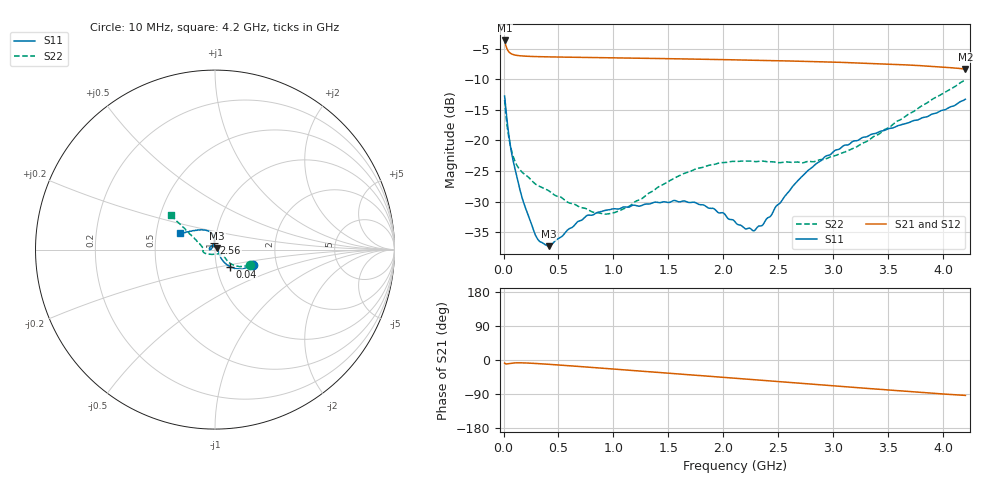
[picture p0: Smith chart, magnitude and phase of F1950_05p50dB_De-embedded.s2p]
! Integrated Device Technology
! Corporate Headquarters
! 6024 Silver Creek Valley Road
! San Jose, CA 95138  USA
! Phone:  1-408-284-8200
! Toll Free:  1-800-223-1366
! Webpage:  http://www.idt.com/
! Timing and RF Division
! 515 Groton Road, Suite 102
! Westford, MA 01886-6024
! Device:  F1950
! Description: 7-bit 0.25 dB Digital Step Attenuator
! Frequency:  150.0 -  4000.00 MHz
! Package:  4x4 mm Thin QFN Plastic Package: 24 pin
! Ports:  2 RF, 12 DC
!  Pin  1  = D0
!  Pin  2  = VDD
!  Pin  3  = Vmode
!  Pin  4  = GND
!  Pin  5  = RF1  =  Port 1
!  Pin  6  = GND
!  Pin  7  = GND
!  Pin  8  = GND
!  Pin  9  = GND
!  Pin 10  = GND
!  Pin 11  = GND
!  Pin 12  = GND
!  Pin 13  = GND
!  Pin 14  = RF2  =  Port 2
!  Pin 15  = GND
!  Pin 16  = LE
!  Pin 17  = CLK
!  Pin 18  = DATE
!  Pin 19  = D6
!  Pin 20  = D5
!  Pin 21  = D4
!  Pin 22  = D3
!  Pin 23  = D2
!  Pin 24  = D1
! State:  22
! Atten State:  5.50 dB
! Voltage:  +5.00 Volts
! Current:  Not Measured mA
! Data:  The device was measured on a the F195X evaluation board which has
!  individual transmission lines to the RF pins.  Data was collected
!  using a calibrated network analyzer.  The evaluation board was
!  de-embedded using a TRL calibration technique.
!  The reference plane is the edge of the package pin.
! Misc:  Board 2019
!  Action Tracker AT0250
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# GHz S dB R 50
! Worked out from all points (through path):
!   420 points, 10 MHz to 4.2 GHz, reference 50 ohm
!   highest |S21| = -3.69 dB at 10 MHz (marker M1); lowest = -8.3 dB at 4.2 GHz (marker M2)
!   group delay of S21, straight-line fit = 60.3 ps
!   lowest |S11| = -37.2 dB at 410 MHz (marker M3), VSWR 1.03, Z = 51.2 + j0.769 ohm
!   |S11| at or under -10 dB: start of sweep to end of sweep
!   |S22| runs from -32.0 to -10.1 dB; largest |S21 - S12| = 0.00071
!   S11 on the Smith chart (normalised r, x): 10 MHz: 1.51, -0.28; 40 MHz: 1.16, -0.22; 2.56 GHz: 0.99, +0.07; 4.2 GHz: 0.66, +0.13
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0.01  -12.75 -22.0  -3.69 -8.2  -3.69 -8.2  -13.39 -24.5
0.04  -17.97 -48.4  -5.33 -9.9  -5.33 -9.9  -18.60 -42.0
0.07  -21.69 -54.6  -5.85 -8.4  -5.85 -8.4  -21.44 -41.5
0.1  -24.29 -55.0  -6.05 -7.6  -6.05 -7.6  -23.20 -38.1
0.19  -30.51 -39.9  -6.24 -7.7  -6.24 -7.7  -25.50 -36.8
0.31  -36.08 -6.1  -6.33 -9.5  -6.32 -9.5  -27.33 -37.1
0.41  -37.24 33.1  -6.36 -11.3  -6.36 -11.3  -28.17 -38.3
0.71  -33.00 97.9  -6.45 -17.5  -6.45 -17.5  -30.95 -56.5
0.91  -31.47 117.8  -6.50 -21.9  -6.50 -21.9  -31.98 -80.6
1  -31.15 125.1  -6.52 -23.8  -6.52 -23.8  -31.81 -95.1
1.14  -30.86 138.0  -6.56 -26.8  -6.56 -26.8  -30.76 -115.7
1.41  -30.12 160.9  -6.63 -32.8  -6.63 -32.8  -27.56 -142.1
1.74  -30.10 179.3  -6.73 -40.0  -6.73 -40.0  -24.68 -159.0
2  -31.82 177.7  -6.81 -45.8  -6.81 -45.8  -23.60 -167.3
2.11  -33.37 171.1  -6.85 -48.3  -6.85 -48.3  -23.42 -170.2
2.28  -34.71 138.7  -6.91 -52.0  -6.91 -52.0  -23.43 -173.7
2.36  -33.73 122.9  -6.95 -53.8  -6.94 -53.8  -23.36 -175.5
2.56  -29.05 97.9  -7.02 -58.2  -7.02 -58.2  -23.51 179.8
2.81  -24.33 93.1  -7.13 -63.8  -7.13 -63.8  -23.46 172.8
3.09  -20.87 100.1  -7.27 -70.1  -7.27 -70.1  -21.98 164.7
3.51  -18.04 119.2  -7.55 -79.4  -7.54 -79.5  -17.82 151.9
4.2  -13.27 155.1  -8.35 -93.4  -8.35 -93.5  -10.12 142.2
